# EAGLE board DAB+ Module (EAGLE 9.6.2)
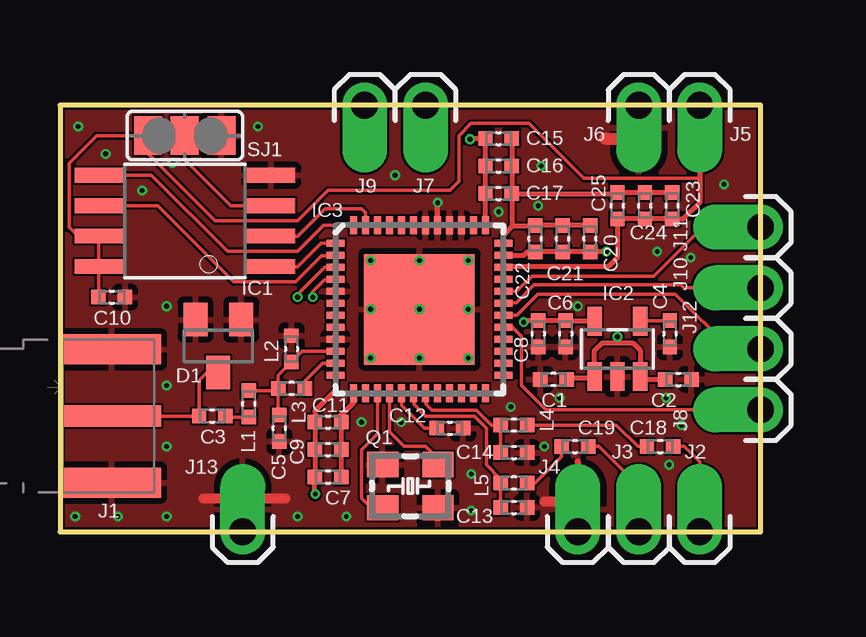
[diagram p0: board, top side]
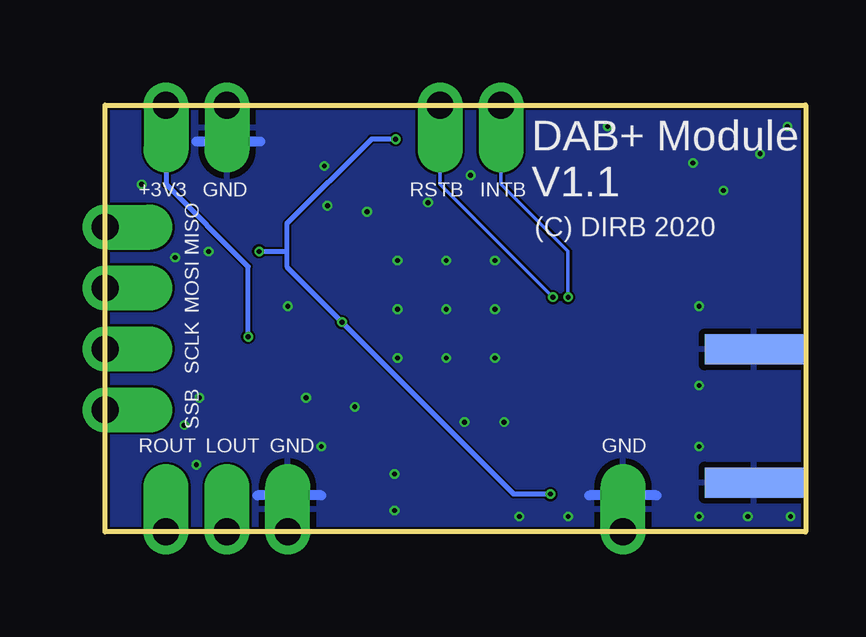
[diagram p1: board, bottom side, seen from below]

Size 29.21 x 17.78 mm. Coordinates in mm from the lower left corner, seen from the top.
Outline: 0,0 29.21,0 29.21,17.78 0,17.78 0,0
Copper layers (1*16): Top 0.035mm / dielectric 0.2mm / Bottom 0.035mm
Design rules "jlcpcb-2-layer": minimum track width 3.5mil, minimum drill 0.2mm, track to track 3.5mil, track to pad 5mil, pad to pad 5mil, via to via 5mil, smd to smd 0mil, copper to edge 0.1mm, drill to drill 5mil, minimum pad ring 4mil, minimum via ring 4mil, stop-mask expansion 3mil, vias tented up to drill 100mil, thermal gap 10mil

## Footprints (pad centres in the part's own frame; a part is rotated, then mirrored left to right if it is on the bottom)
SMD0402 = smd 0.6 x 0.6: 1 -0.55,0; 2 0.55,0
SOT23C = smd 1 x 1.4: 1 -0.95,-1.1; 2 0.95,-1.1; 3 0,1.1
SO08 = smd 0.61 x 2: 1 -1.905,-3.6; 2 -0.635,-3.6; 3 0.635,-3.6; 4 1.905,-3.6; 5 1.905,3.6; 6 0.635,3.6; 7 -0.635,3.6; 8 -1.905,3.6
SOT23-5 = smd 0.6 x 1.2: 1 -0.95,-1.15; 2 0,-1.15; 3 0.95,-1.15; 4 0.95,1.15; 5 -0.95,1.15
QFN48 = smd 0.75 x 0.3: 1 -3.5,2.75; 2 -3.5,2.25; 3 -3.5,1.75; 4 -3.5,1.25; 5 -3.5,0.75; 6 -3.5,0.25; 7 -3.5,-0.25; 8 -3.5,-0.75; 9 -3.5,-1.25; 10 -3.5,-1.75; 11 -3.5,-2.25; 12 -3.5,-2.75; 25 3.5,-2.75; 26 3.5,-2.25; 27 3.5,-1.75; 28 3.5,-1.25; 29 3.5,-0.75; 30 3.5,-0.25; 31 3.5,0.25; 32 3.5,0.75; 33 3.5,1.25; 34 3.5,1.75; 35 3.5,2.25; 36 3.5,2.75 | smd 0.3 x 0.75: 13 -2.75,-3.5; 14 -2.25,-3.5; 15 -1.75,-3.5; 16 -1.25,-3.5; 17 -0.75,-3.5; 18 -0.25,-3.5; 19 0.25,-3.5; 20 0.75,-3.5; 21 1.25,-3.5; 22 1.75,-3.5; 23 2.25,-3.5; 24 2.75,-3.5; 37 2.75,3.5; 38 2.25,3.5; 39 1.75,3.5; 40 1.25,3.5; 41 0.75,3.5; 42 0.25,3.5; 43 -0.25,3.5; 44 -0.75,3.5; 45 -1.25,3.5; 46 -1.75,3.5; 47 -2.25,3.5; 48 -2.75,3.5 | smd 4.6 x 4.6: EP 0,0
60312202114508 = smd 0.9 x 4.1: 1 0,0 | smd 1.25 x 4.1: 2 -2.775,0; 3 2.775,0 | smd 1.25 x 4.1 bottom: 4 -2.775,0; 5 2.775,0
1X01_OFFSET = drill 1.118 pad 1.88 offset: 1 0,0
XTAL_3.2X2.5 = smd 1.3 x 1.05: 1 -1.15,-0.9; 2 1.15,-0.9; 3 1.15,0.9; 4 -1.15,0.9
SJ_2 = smd 1.168 x 1.6: 1 -1.524,0; 2 0,0; 3 1.524,0

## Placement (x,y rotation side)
C1  2.2u  [SMD0402]  20.57,6.35 180 top
C2  100n  [SMD0402]  25.78,6.35 0 top
C3  33p  [SMD0402]  6.35,4.83 0 top
C4  10n  [SMD0402]  25.43,8.26 270 top
C5  2.7p  [SMD0402]  9.14,4.32 90 top
C6  100n  [SMD0402]  21.08,8.26 270 top
C7  1u  [SMD0402]  11.18,2.29 0 top
C8  2.2u  [SMD0402]  19.94,8.26 270 top
C9  2.2n  [SMD0402]  11.18,3.43 0 top
C10  2.2n  [SMD0402]  2.16,9.78 0 top
C11  8.2p  [SMD0402]  11.18,4.57 0 top
C12  1u  [SMD0402]  16.26,4.32 0 top
C13  8.2p  [SMD0402]  18.92,1.02 0 top
C14  8.2p  [SMD0402]  18.92,3.3 0 top
C15  1u  [SMD0402]  18.29,16.38 0 top
C16  2.2n  [SMD0402]  18.29,15.24 0 top
C17  8.2p  [SMD0402]  18.29,14.1 0 top
C18  1u  [SMD0402]  25.02,3.56 0 top
C19  1u  [SMD0402]  21.46,3.56 0 top
C20  1u  [SMD0402]  22.1,12.22 90 top
C21  2.2n  [SMD0402]  20.95,12.22 90 top
C22  8.2p  [SMD0402]  19.81,12.22 90 top
C23  1u  [SMD0402]  25.53,13.59 90 top
C24  2.2n  [SMD0402]  24.38,13.59 90 top
C25  8.2p  [SMD0402]  23.24,13.59 90 top
D1  BAV99  [SOT23C]  6.6,7.75 180 top
IC1  SST25VF016B  [SO08]  5.21,12.95 90 top
IC2  TPS79318DBVR  [SOT23-5]  23.24,7.62 0 top
IC3  SI4684-A10-GM  [QFN48]  14.99,9.27 0 top
J1  SMA PCB 1.1mm  [60312202114508]  2.16,4.83 270 top
J2  [1X01_OFFSET]  26.67,0 0 top
J3  [1X01_OFFSET]  24.13,0 0 top
J4  [1X01_OFFSET]  21.59,0 0 top
J5  [1X01_OFFSET]  26.67,17.78 180 top
J6  [1X01_OFFSET]  24.13,17.78 180 top
J7  [1X01_OFFSET]  15.24,17.78 180 top
J8  [1X01_OFFSET]  29.21,5.08 90 top
J9  [1X01_OFFSET]  12.7,17.78 180 top
J10  [1X01_OFFSET]  29.21,10.16 90 top
J11  [1X01_OFFSET]  29.21,12.7 90 top
J12  [1X01_OFFSET]  29.21,7.62 90 top
J13  [1X01_OFFSET]  7.62,0 0 top
L1  18nH  [SMD0402]  7.87,5.33 90 top
L2  120nH  [SMD0402]  9.65,7.62 270 top
L3  22nH  [SMD0402]  9.65,5.97 180 top
L4  BLM15HG102SN1D  [SMD0402]  18.92,4.45 180 top
L5  BLM15HG102SN1D  [SMD0402]  18.92,2.03 180 top
Q1  19.2MHz  [XTAL_3.2X2.5]  14.61,1.91 0 top
SJ1  [SJ_2]  5.21,16.51 180 top

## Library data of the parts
C1-C25 L1-L5 Q1 = generisch
D1 = semicon-smd-ipc
IC1 = sst25
IC2 = ldo_reg
IC3 = SI4688-A10-GM
J1 = Wurth_Connectors_WR-SMA; DATASHEET-URL: https://www.we-online.com/catalog/datasheet/60312202114508.pdf; GENDER: Jack; INTERFACE: MIL-STD-348; MOUNT: End Launch; ORIENTATION-TYPE: Straight; PART-NUMBER: 60312202114508; Z: 50Ohm
J2-J13 = SparkFun-Connectors
SJ1 = jumper

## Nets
+1V8: C6.1 C7.1 C8.1 C9.1 C11.1 C15.1 C16.1 C17.1 C20.1 C21.1 C22.1 IC2.5 IC3.12 IC3.35 IC3.37
+3V3: C1.1 C2.1 C10.1 C23.1 C24.1 C25.1 IC1.7 IC1.8 IC2.1 IC2.3 IC3.34 J5.1 SJ1.3
ABYP: C7.2 C9.2 C11.2 IC3.13
AMLOOPN: IC3.6
AMLOOPP: IC3.7
DBYP: C15.2 C16.2 C17.2 C20.2 C21.2 C22.2 C23.2 C24.2 C25.2 IC3.36
GND: C1.2 C2.2 C4.2 C5.1 C6.2 C8.2 C10.2 C12.2 C13.2 C14.2 D1.1 D1.2 IC1.4 IC2.2 IC3.5 IC3.9 IC3.39 IC3.40 IC3.41 IC3.42 IC3.EP J1.2 J1.3 J1.4 J1.5 J4.1 J6.1 J13.1 L2.1 Q1.2 Q1.4 SJ1.1
INTB_SI: IC3.3 J9.1
LOUT: C19.2 J3.1
MISO_FLASH: IC1.2 IC3.47
MISO_SI: IC3.32 J11.1
MOSI_FLASH: IC1.5 IC3.48
MOSI_SI: IC3.31 J10.1
N$1: C3.2 L1.1
N$2: C5.2 IC3.10 L1.2 L2.2 L3.2
N$3: IC3.11 L3.1
N$4: C18.1 L4.1
N$5: C19.1 L5.1
N$6: IC3.15 Q1.1
N$7: IC3.16 Q1.3
N$8: C12.1 IC3.17
N$9: IC1.3 SJ1.2
N$11: C4.1 IC2.4
RF_IN: C3.1 D1.3 J1.1
ROUT: C18.2 J2.1
RSTB_SI: IC3.4 J7.1
SCK_FLASH: IC1.6 IC3.2
SCLK_SI: IC3.30 J12.1
SI4688_LOUT: C13.1 IC3.18 L5.2
SI4688_ROUT: C14.1 IC3.19 L4.2
SSB_FLASH: IC1.1 IC3.1
SSB_SI: IC3.29 J8.1
WHIP: IC3.8

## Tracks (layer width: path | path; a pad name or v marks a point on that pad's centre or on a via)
+1V8  (via drill 0.2 pad 0.23)
  Top 0.203: IC3.37 C17.1 C16.1 C15.1 17.12,16.38 v17.09,16.36 | IC3.35 19.34,11.52 19.48,11.67 C22.1 C21.1 C20.1 22.77,11.67 v22.78,11.68 | IC3.12 11.49,5.9 10.63,5.04 C11.1 C9.1 C7.1 10.59,2.25 10.59,1.63 v10.64,1.57 | IC2.5 21.12,8.77 C6.1 C8.1 19.4,8.8 v19.33,8.74
  Bottom 0.203: v17.09,16.36 18.11,16.36 21.64,12.83 21.64,11.68 | 21.64,11.68 21.64,11.05 v19.33,8.74 12.17,1.57 v10.64,1.57 | v22.78,11.68 21.64,11.68
+3V3  (via drill 0.2 pad 0.23)
  Top 0.15: C10.1 IC1.8 IC1.7 0.76,12.32 0.38,12.7 0.38,15.37 1.52,16.51 SJ1.3 3.68,15.75 6.48,12.95 9.91,12.95 11.18,14.22 16.26,14.22 16.64,14.61 16.64,16.51 17.14,17.02 19.56,17.02 21.84,14.73 26.67,14.73
  Top 0.2: J5.1 26.67,14.73 26.67,13.72 25.99,13.04 C23.1 | 23.24,7.87 22.61,7.87 22.29,7.56 IC2.1 22.21,6.39 21.17,6.39 C1.1 | 23.24,7.87 23.88,7.87 24.19,7.56 IC2.3 24.32,6.34 C2.1 | 23.24,7.87 v23.24,8.13
  Top 0.203: C23.1 C24.1 C25.1 23.24,11.43 22.86,11.05 18.51,11.05 IC3.34
  Bottom 0.2: v23.24,8.13 23.24,11.05 26.67,14.48 J5.1
ABYP
  Top 0.203: IC3.13 12.24,5.38 11.68,4.83 11.68,4.61 C11.2 C9.2 C7.2
DBYP
  Top 0.203: C15.2 C16.2 C17.2 | C17.2 23.2,14.1 C25.2 C24.2 C23.2 | 18.85,12.72 19.77,12.72 C22.2 C21.2 C20.2 | 18.85,12.72 18.49,12.37 IC3.36 | C17.2 18.84,12.73 18.85,12.72
GND  (via drill 0.2 pad 0.23)
  Top 0.203: IC3.41 15.74,13.7 v15.75,13.72
  Top 0.254: 21.59,2.92 21.59,1.27 J4.1
  Top 0.406: 7.62,1.4 9.4,1.4 | J13.1 7.62,1.4 | 5.97,1.4 7.62,1.4 | 21.46,1.27 21.59,1.14 J4.1 | 20.19,1.27 21.59,1.27
  Top 0.508: 22.73,16.38 24,16.38 24.13,16.51 J6.1
  Bottom 0.406: 6.22,1.52 7.62,1.52 | J13.1 7.62,1.52 | 7.62,1.52 9.02,1.52 | 20.19,1.52 21.59,1.52 | J4.1 21.59,1.52 | 22.73,16.26 24.13,16.26 | J6.1 24.13,16.26 | 24.13,16.26 25.4,16.26 | 21.59,1.52 22.86,1.52
  other vias: 20.19,3.56 12.95,11.3 17.02,11.3 17.02,7.24 12.95,7.24 12.95,9.27 17.02,9.27 14.99,11.3 14.99,7.24 14.99,9.27 12.57,4.57 18.8,5.21 20.07,15.24 19.94,13.59 27.69,14.48 26.29,11.43 25.4,2.79 25.91,4.45 21.59,9.4 0.76,16.89 1.91,15.75 3.43,14.22 4.7,15.37 8.26,16.89 4.45,6.1 4.45,3.56 4.45,9.4 4.45,0.64 2.41,0.64 0.64,0.64 9.91,0.64 11.94,0.64 17.14,2.41 17.14,0.89 20.83,5.59 25.27,5.59 13.97,14.86 18.29,13.34 14.22,4.57 24.89,11.68
  pour Top: 0.13,17.78 29.21,17.78 29.21,0 0,0 0,17.78
  pour Bottom: 0,17.78 29.21,17.78 29.21,0 0,0
INTB_SI  (via drill 0.2 pad 0.23)
  Top 0.15: IC3.3 11.02,11.02 9.91,9.91 v9.91,9.78
  Bottom 0.15: J9.1 12.7,14.48 9.91,11.68 v9.91,9.78
LOUT
  Top 0.15: C19.2 22.48,3.56 24.13,1.91 J3.1
MISO_FLASH
  Top 0.15: IC3.47 12.74,13.3 12.57,13.46 11.05,13.46 9.91,12.32 IC1.2
MISO_SI
  Top 0.15: J11.1 26.8,12.7 24.75,10.66 19.67,10.66 19.04,10.02 IC3.32
MOSI_FLASH
  Top 0.15: IC3.48 10.99,12.77 9.91,11.68 6.99,11.68 3.81,14.86 IC1.5
MOSI_SI
  Top 0.15: IC3.31 18.51,9.54 19.02,9.54 19.77,10.29 25.89,10.29 26.01,10.16 J10.1
N$1
  Top 0.15: L1.1 6.94,4.78 C3.2
N$2
  Top 0.15: IC3.10 10.1,7.52 L2.2 9.1,6.52 L3.2 | C5.2 9.1,4.91 L3.2 | L1.2 9.02,5.88 L3.2 | L3.2
N$3
  Top 0.15: IC3.11 10.96,7.02 10.2,6.26 L3.1
N$4
  Top 0.15: C18.1 24.09,3.56 23.2,4.45 L4.1
N$5
  Top 0.15: C19.1 20.91,3.13 19.81,2.03 L5.1
N$6
  Top 0.15: IC3.15 13.24,4.09 12.57,3.43 12.57,1.4 12.96,1 Q1.1
N$7
  Top 0.15: IC3.16 13.74,4.17 14.35,3.56 15.24,3.56 15.76,3.04 Q1.3
N$8
  Top 0.15: IC3.17 14.24,5.28 15.2,4.32 C12.1
N$9
  Top 0.15: IC1.3 7.11,13.59 5.21,15.49 SJ1.2
N$11
  Top 0.15: IC2.4 24.16,8.8 C4.1
RF_IN
  Top 0.15: D1.3 6.14,6.65 5.8,6.31 C3.1 J1.1
ROUT
  Top 0.15: C18.2 26.04,3.56 26.67,2.92 J2.1
RSTB_SI  (via drill 0.2 pad 0.23)
  Top 0.15: IC3.4 11.46,10.5 11.03,10.5 10.54,10.01 v10.54,9.78
  Bottom 0.15: v10.54,9.78 15.24,14.48 J7.1
SCK_FLASH
  Top 0.15: IC3.2 11.46,11.5 10.9,11.5 9.81,10.41 7.24,10.41 4.06,13.59 IC1.6
SCLK_SI
  Top 0.15: IC3.30 19.04,9.02 19.93,9.91 25.65,9.91 27.94,7.62 J12.1
SI4688_LOUT
  Top 0.15: IC3.18 14.76,5.75 14.76,5.31 15.24,4.83 17.27,4.83 17.78,4.32 17.78,2.79 18.37,2.2 L5.2 C13.1
SI4688_ROUT
  Top 0.15: IC3.19 15.26,5.75 15.26,5.31 15.5,5.07 17.37,5.07 17.99,4.45 L4.2 C14.1
SSB_FLASH
  Top 0.15: IC3.1 10.88,12.02 9.91,11.05 IC1.1
SSB_SI
  Top 0.15: J8.1 20.27,5.08 19.24,6.11 19.24,8.15 18.87,8.52 IC3.29

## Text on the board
bNames: DAB+ Module / V1.1 | INTB | RSTB | GND | MISO | +3V3 | (C) DIRB 2020 | MOSI | SCLK | SSB | GND | GND | LOUT | ROUT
